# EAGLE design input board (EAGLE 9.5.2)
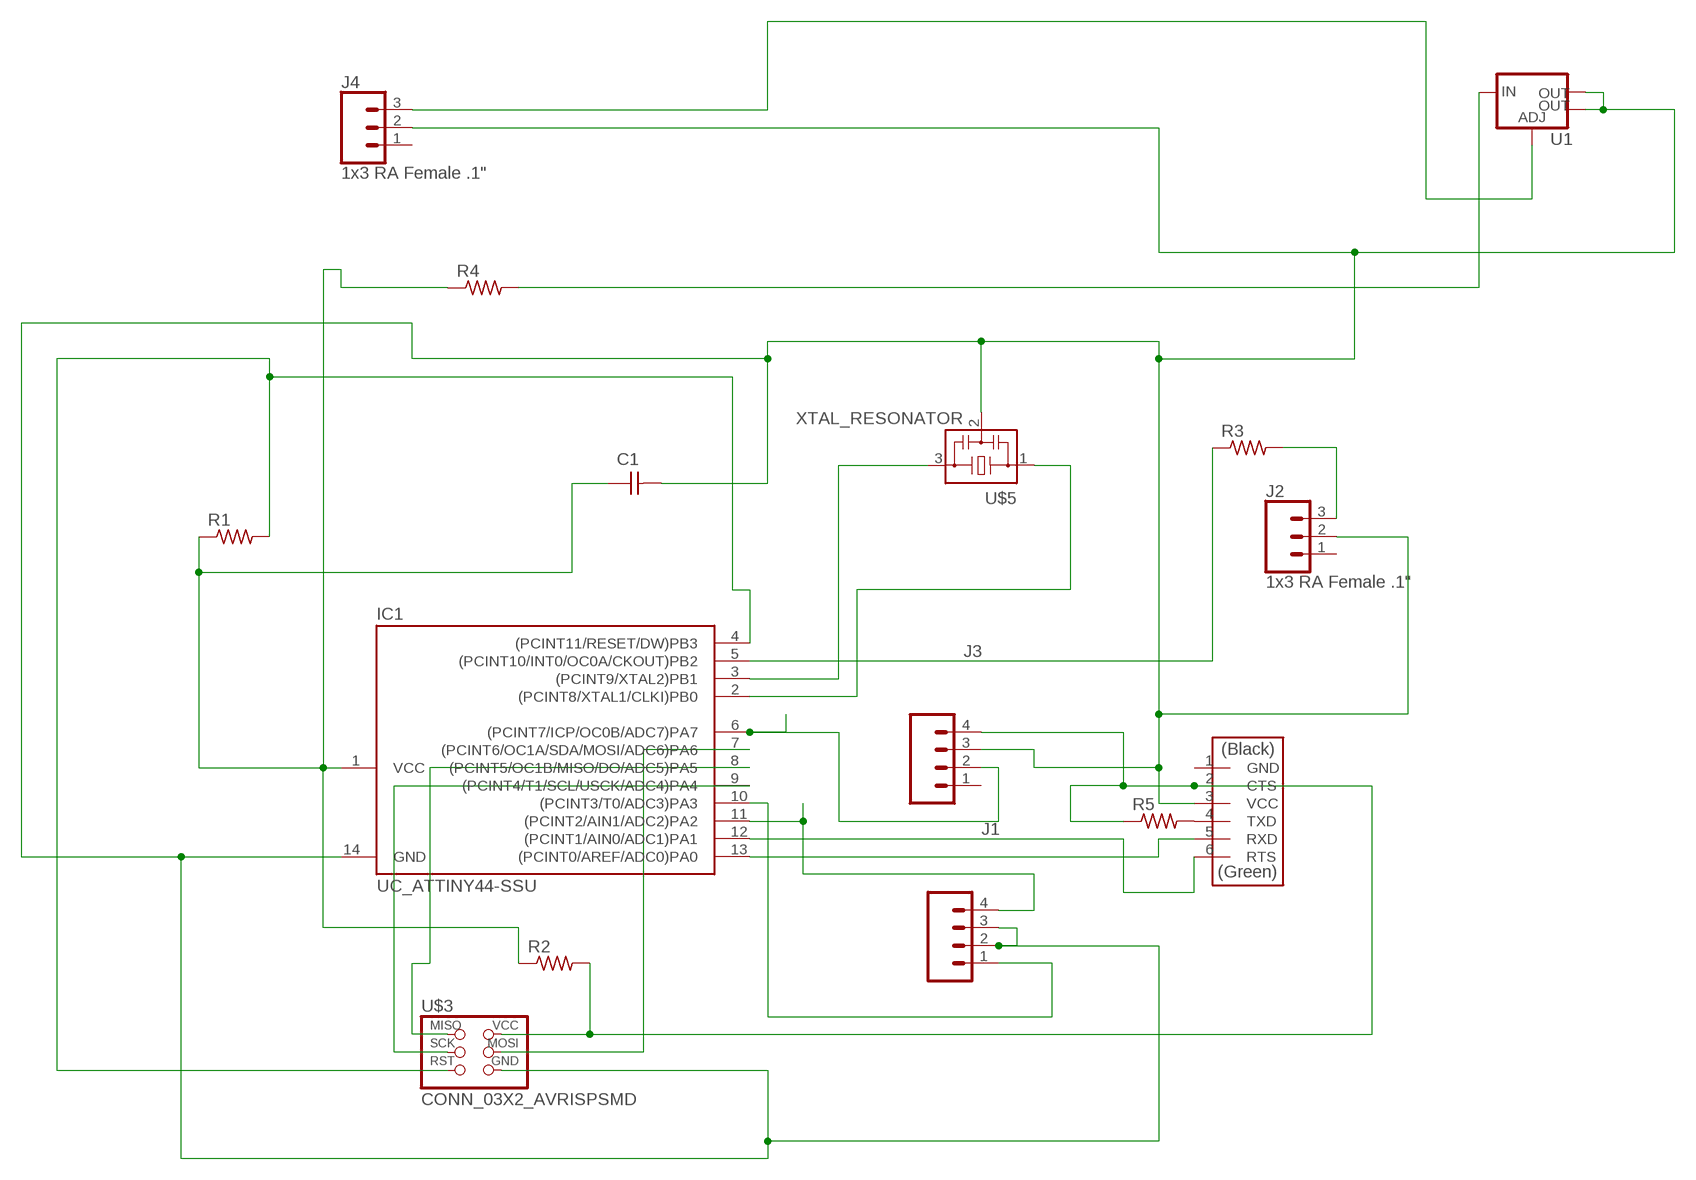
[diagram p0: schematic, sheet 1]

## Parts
C1  CAP_UNPOLARIZEDFAB  [C1206FAB]
IC1  UC_ATTINY44-SSU  [SOIC14]
J1  CONN_04SMD_RA_FEMALE  [1X04_SMD_RA_FEMALE]
J2  1x3 RA Female .1"  CONN_03SMD_RA_FEMALE  [1X03_SMD_RA_FEMALE]
J3  CONN_04SMD_RA_FEMALE  [1X04_SMD_RA_FEMALE]
J4  1x3 RA Female .1"  CONN_03SMD_RA_FEMALE  [1X03_SMD_RA_FEMALE]
R1  R1206  [R1206]
R2  R1206  [R1206]
R3  R1206FAB  [R1206FAB]
R4  R1206  [R1206]
R5  R1206  [R1206]
U1  VR_REGULATOR_LM1117SOT223  [SOT223]
U$2  CONN_06_FTDI-SMD-HEADER  [1X06SMD]
U$3  CONN_03X2_AVRISPSMD  [2X03SMD]
U$5  XTAL_RESONATOR  [EFOBM]

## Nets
N$1: R5.2 U$2.4(TXD)
N$2: IC1.4((PCINT11/RESET/DW)PB3) R1.2 U$3.5(RST)
N$3: IC1.6((PCINT7/ICP/OC0B/ADC7)PA7) J3.2
N$4: IC1.5((PCINT10/INT0/OC0A/CKOUT)PB2) R3.1
N$5: IC1.2((PCINT8/XTAL1/CLKI)PB0) U$5.1
N$6: IC1.3((PCINT9/XTAL2)PB1) U$5.3
N$7: J4.3 U1.1(ADJ)
N$8: R4.2 U1.3(IN)
N$9: J2.3 R3.2
N$10: IC1.9((PCINT4/T1/SCL/USCK/ADC4)PA4) U$3.3(SCK)
N$11: IC1.8((PCINT5/OC1B/MISO/DO/ADC5)PA5) U$3.1(MISO)
N$12: IC1.7((PCINT6/OC1A/SDA/MOSI/ADC6)PA6) U$3.4(MOSI)
N$13: IC1.11((PCINT2/AIN1/ADC2)PA2) J1.4
N$14: IC1.12((PCINT1/AIN0/ADC1)PA1) U$2.6(RTS)
N$15: IC1.13((PCINT0/AREF/ADC0)PA0) U$2.5(RXD)
N$16: IC1.10((PCINT3/T0/ADC3)PA3) J1.1
N$17: C1.1 IC1.1(VCC) R1.1 R2.1 R4.1
N$18: C1.2 IC1.14(GND) J1.2 J1.3 J2.2 J3.3 J4.2 U1.2(OUT) U1.4(OUT) U$2.3(VCC) U$3.6(GND) U$5.2
N$19: J3.4 R2.2 R5.1 U$2.2(CTS) U$3.2(VCC)
Unconnected: J2.1 J3.1 J4.1 U$2.1(GND)

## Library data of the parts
C1 = fab:CAP_UNPOLARIZED
IC1 = fab:UC_ATTINY44
J1 J3 = SparkFun-Connectors:CONN_04: Multi connection point. Often used as Generic Header-pin footprint for 0.1 inch spaced/style header connections On any of the 0.1 inch spaced packages, you can populate with these: Break Away Headers - Straight (PRT-00116) Break Away Male Headers - Right Angle (PRT-00553) Female Headers (PRT-00115)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; PROD_ID: CONN-12382
J2 J4 = SparkFun-Connectors:CONN_03: Multi connection point. Often used as Generic Header-pin footprint for 0.1 inch spaced/style header connections On any of the 0.1 inch spaced packages, you can populate with these: Break Away Headers - Straight (PRT-00116) Break Away Male Headers - Right Angle (PRT-00553) Female Headers (PRT-00115)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; PROD_ID: CONN-10926
R1-R5 = fab:R: Resistor (US Symbol)
U1 = fab:VR_REGULATOR_LM1117: Voltage Regulator LM1117 Standard adjustable voltage regulator but in SMD form. Spark Fun Electronics SKU : COM-00595; PROD_ID: VREG-08170
U$2 = fab:CONN_06_FTDI-SMD-HEADER
U$3 = fab:CONN_03X2_AVRISP
U$5 = fab:XTAL_RESONATOR

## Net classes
0 default: width 0.203 mm, clearance 0.508 mm

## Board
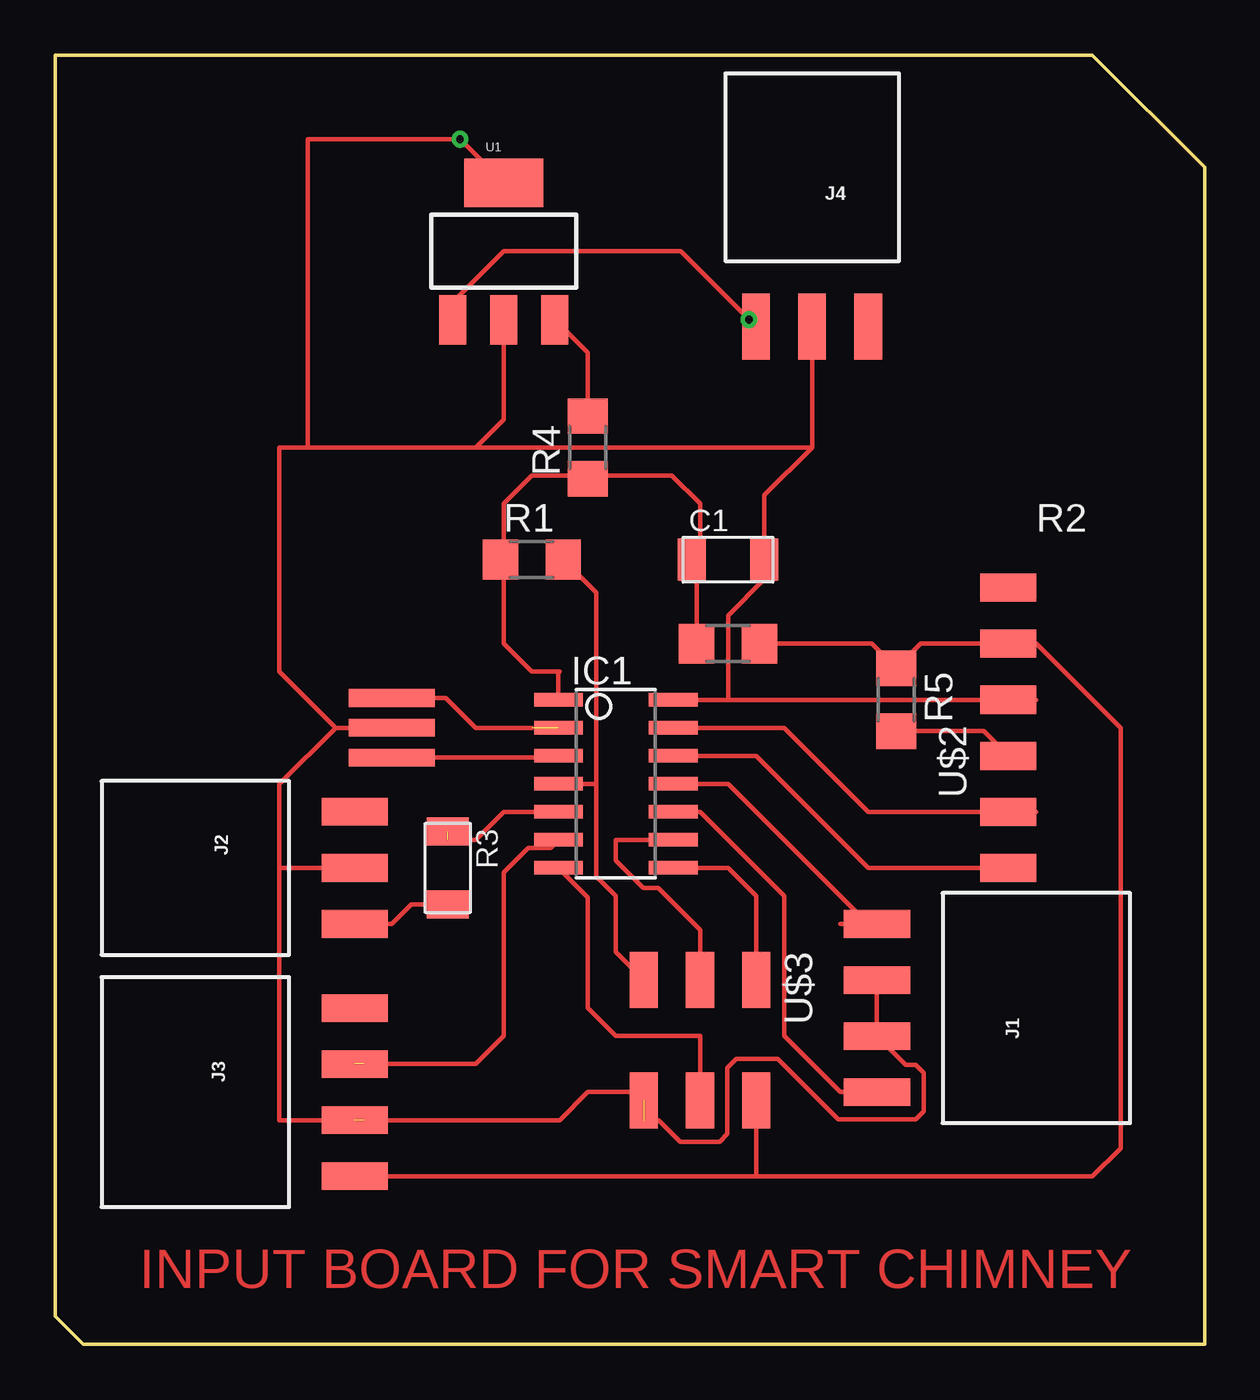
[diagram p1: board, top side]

Size 52.07 x 58.42 mm. Coordinates in mm from the lower left corner, seen from the top.
Outline: 0,58.42 46.99,58.42 52.07,53.34 52.07,0 1.27,0 0,1.27 0,58.42
Copper layers (1*16): Top 0.035mm / dielectric 1.5mm / Bottom 0.035mm
Design rules "input board": minimum track width 6mil, minimum drill 0.35mm, track to track 0.205mm, track to pad 0.205mm, pad to pad 0.205mm, via to via 0.205mm, smd to smd 6mil, copper to edge 40mil, drill to drill 6mil, minimum pad ring 10mil, minimum via ring 8mil, stop-mask expansion 4mil, vias tented up to drill 0mil, thermal gap 10mil

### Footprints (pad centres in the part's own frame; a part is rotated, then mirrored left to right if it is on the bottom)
C1206FAB = smd 1.27 x 1.905: 1 -1.651,0; 2 1.651,0
SOIC14 = smd 0.61 x 2.21: 1 -3.81,-2.603; 2 -2.54,-2.603; 3 -1.27,-2.603; 4 0,-2.603; 5 1.27,-2.603; 6 2.54,-2.603; 7 3.81,-2.603; 8 3.81,2.603; 9 2.54,2.603; 10 1.27,2.603; 11 0,2.603; 12 -1.27,2.603; 13 -2.54,2.603; 14 -3.81,2.603
1X04_SMD_RA_FEMALE = smd 1.25 x 3: 1 -3.81,7.225; 2 -1.27,7.225; 3 1.27,7.225; 4 3.81,7.225
1X03_SMD_RA_FEMALE = smd 1.25 x 3: 1 -2.54,7.225; 2 0,7.225; 3 2.54,7.225
R1206 = smd 1.6 x 1.803: 1 -1.422,0; 2 1.422,0
R1206FAB = smd 1.27 x 1.905: 1 -1.651,0; 2 1.651,0
SOT223 = smd 1.219 x 2.235: 1 -2.311,-3.099; 2 0,-3.099; 3 2.311,-3.099 | smd 3.6 x 2.2: 4 0,3.099
1X06SMD = smd 2.54 x 1.27: 1 0,6.35; 2 0,3.81; 3 0,1.27; 4 0,-1.27; 5 0,-3.81; 6 0,-6.35
2X03SMD = smd 2.54 x 1.27: 1 -2.54,2.54; 2 2.92,2.54; 3 -2.54,0; 4 2.92,0; 5 -2.54,-2.54; 6 2.92,-2.54
EFOBM = smd 0.8 x 3.9: 1 -1.35,0; 2 0,0; 3 1.35,0

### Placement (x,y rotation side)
C1  30.48,35.56 0 top
IC1  25.4,25.4 270 top
J1  44.45,15.24 90 top
J2  6.35,21.59 270 top
J3  6.35,11.43 270 top
J4  34.29,53.34 180 top
R1  21.59,35.56 0 top
R2  30.48,31.75 0 top
R3  17.78,21.59 270 top
R4  24.13,40.64 90 top
R5  38.1,29.21 270 top
U1  20.32,49.53 0 top
U$2  43.18,27.94 0 top
U$3  29.21,13.97 270 top
U$5  15.24,27.94 270 top

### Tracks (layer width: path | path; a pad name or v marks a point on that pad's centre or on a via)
N$1
  Top 0.203: R5.2 42.06,27.79 U$2.4
N$2
  Top 0.203: U$3.5 25.4,17.78 25.4,20.32 24.51,21.21 24.51,25.4 | R1.2 24.51,34.06 24.51,25.4 | IC1.4 24.51,25.4
N$3  (1 unrouted)
  Top 0.203: IC1.6 22.44,22.5 21.44,22.5 20.32,21.38 20.32,13.97 19.05,12.7 13.97,12.7
N$4  (1 unrouted)
  Top 0.203: IC1.5 20.32,24.13 19.05,22.86 17.78,22.86
N$5  (1 unrouted)
  Top 0.203: U$5.1 17.7,29.29 19.05,27.94 21.59,27.94
N$6
  Top 0.203: U$5.3 22.72,26.59 IC1.3
N$7  (via drill 0.35)
  Top 0.203: v31.43,46.43 J4.3 28.34,49.53 20.32,49.53 18.01,47.22 U1.1
N$8
  Top 0.203: R4.2 24.13,44.93 U1.3
N$9
  Top 0.203: R3.2 16.13,19.94 15.24,19.05 J2.3
N$10
  Top 0.203: U$3.3 29.21,18.79 27.32,20.68 26.65,20.68 25.4,21.92 25.4,22.86 IC1.9
N$11
  Top 0.203: IC1.8 30.48,21.59 31.75,20.32 U$3.1
N$12
  Top 0.203: IC1.7 24.13,20.26 24.13,15.24 25.4,13.97 29.21,13.97 U$3.4
N$13
  Top 0.203: IC1.11 30.48,25.4 36.83,19.05 | 35.56,19.05 36.83,19.05 | 36.83,19.05 J1.4
N$14
  Top 0.203: IC1.12 31.75,26.67 36.83,21.59 U$2.6
N$15
  Top 0.203: IC1.13 33.02,27.94 36.83,24.13 U$2.5 44.45,24.13
N$16
  Top 0.203: J1.1 35.56,11.43 33.02,13.97 33.02,20.32 29.21,24.13 IC1.10
N$17
  Top 0.203: 24.13,39.37 27.94,39.37 29.21,38.1 29.21,35.94 C1.1 29.06,35.33 R2.1 | 24.13,39.37 21.59,39.37 20.32,38.1 20.32,35.41 | IC1.1 22.8,30.42 22.86,30.48 21.59,30.48 20.32,31.75 20.32,35.41 | R1.1 20.32,35.41 | R4.1 24.13,39.37
N$18  (via drill 0.35)  (2 unrouted)
  Top 0.203: 30.48,29.21 30.48,33.02 32.13,34.67 C1.2 32.13,38.48 34.29,40.64 | U$5.2 12.7,27.94 | 11.43,40.64 10.16,40.64 10.16,30.48 12.7,27.94 | 11.43,40.64 19.05,40.64 | 19.05,40.64 34.29,40.64 | IC1.14 30.48,29.21 | J1.3 J1.2 38.53,12.66 38.98,12.66 39.34,12.31 39.34,10.55 38.98,10.2 35.47,10.2 32.74,12.93 30.86,12.93 30.45,12.52 30.45,9.53 30.1,9.17 28.32,9.17 27.33,10.16 26.67,10.16 | 12.7,27.94 10.16,25.4 10.16,21.59 | 10.16,21.59 10.16,10.16 13.97,10.16 | J2.2 10.16,21.59 | J3.3 22.86,10.16 24.13,11.43 26.29,11.43 U$3.6 | J4.2 34.29,40.64 | 30.48,29.21 U$2.3 44.45,29.21 | 11.43,40.64 11.43,54.61 v18.34,54.61 U1.4 | 19.05,40.64 20.32,41.91 U1.2
N$19
  Top 0.203: U$3.2 31.75,7.62 | 31.75,7.62 46.99,7.62 48.26,8.89 48.26,27.94 44.45,31.75 U$2.2 39.22,31.75 R5.1 36.98,31.75 R2.2 | J3.4 31.75,7.62

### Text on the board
Top: INPUT BOARD FOR SMART CHIMNEY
